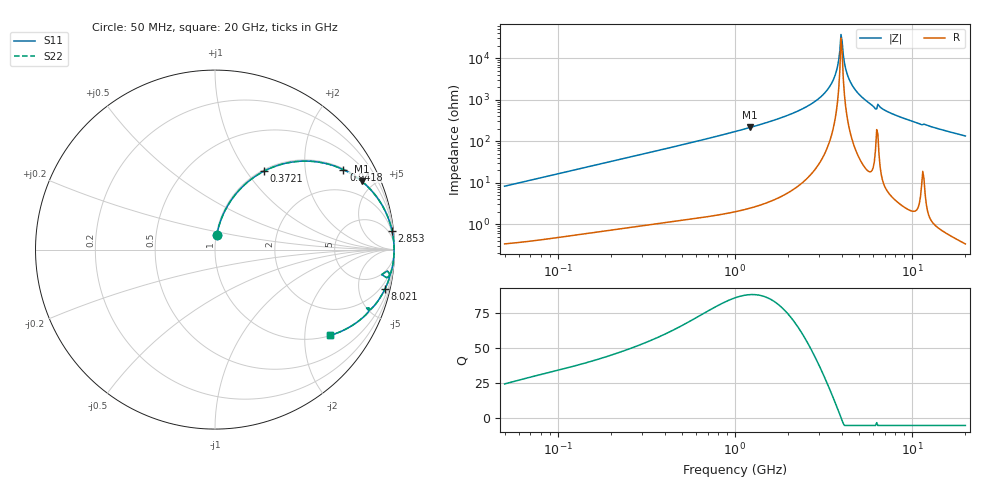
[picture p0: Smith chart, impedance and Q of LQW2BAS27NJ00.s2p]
!Murata Part Number: LQW2BAS27NJ00
!These Parameters are Measured in Series Mode Connection
!  o--[Z]--o
!Port1  Port2
!  o-------o
!Freq. Start=50[MHz] Stop=20[GHz], 401[Steps]
# Hz S RI R 50
!Freq.(Hz) S11(Real) S11(Imag) S21(Real) S21(Imag) S12(Real) S12(Imag) S22(Real) S22(Imag)
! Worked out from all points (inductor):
!   401 points, 50 MHz to 20 GHz, reference 50 ohm
!   read as one part in series: L = 26.1 nH near 51.52 MHz
!   highest Q = 88.1 at 1.215 GHz (marker M1), where L = 28 nH
!   self-resonance near 3.967 GHz
!   S11 on the Smith chart (normalised r, x): 50 MHz: 1.01, +0.16; 372.1 MHz: 1.02, +1.21; 941.8 MHz: 1.04, +3.19; 2.853 GHz: 1, +19; 8.021 GHz: 1.08, -8.56; 20 GHz: 1.01, -2.67
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5e7  0.00999 0.0812  0.99 -0.0812  0.99 -0.0812  0.00999 0.0812
1.364002e8  0.052 0.2095  0.948 -0.2095  0.948 -0.2095  0.052 0.2095
3.721004e8  0.2709 0.4359  0.7291 -0.4359  0.7291 -0.4359  0.2709 0.4359
9.418449e8  0.7157 0.4452  0.2843 -0.4452  0.2843 -0.4452  0.7157 0.4452
1e9  0.742 0.4318  0.258 -0.4318  0.258 -0.4318  0.742 0.4318
1.214974e9  0.8181 0.3801  0.1819 -0.3801  0.1819 -0.3801  0.8181 0.3801
1.962148e9  0.942 0.2272  0.058 -0.2272  0.058 -0.2272  0.942 0.2272
2.728004e9  0.9828 0.1198  0.0172 -0.1198  0.0172 -0.1198  0.9828 0.1198
2.853386e9  0.9862 0.1055  0.0138 -0.1055  0.0138 -0.1055  0.9862 0.1055
3.265178e9  0.9937 0.0627  0.00631 -0.0627  0.00631 -0.0627  0.9937 0.0627
3.572216e9  0.9965 0.0344  0.00346 -0.0344  0.00346 -0.0344  0.9965 0.0344
3.736399e9  0.9973 0.0203  0.00266 -0.0203  0.00266 -0.0203  0.9973 0.0203
3.908127e9  0.9977 0.00621  0.00225 -0.00621  0.00225 -0.00621  0.9977 0.00621
3.967106e9  0.9978 0.0015  0.00221 -0.0015  0.00221 -0.0015  0.9978 0.0015
4.087748e9  0.9977 -0.00793  0.00225 0.00793  0.00225 0.00793  0.9977 -0.00793
4.212059e9  0.9975 -0.0174  0.00248 0.0174  0.00248 0.0174  0.9975 -0.0174
4.34015e9  0.9971 -0.0268  0.00289 0.0268  0.00289 0.0268  0.9971 -0.0268
4.81993e9  0.9942 -0.0602  0.00581 0.0602  0.00581 0.0602  0.9942 -0.0602
6.034176e9  0.9751 -0.1399  0.0249 0.1399  0.0249 0.1399  0.9751 -0.1399
7.442007e9  0.9583 -0.1946  0.0417 0.1946  0.0417 0.1946  0.9583 -0.1946
8.020766e9  0.9465 -0.2206  0.0535 0.2206  0.0535 0.2206  0.9465 -0.2206
2e10  0.641 -0.4785  0.359 0.4785  0.359 0.4785  0.641 -0.4785
